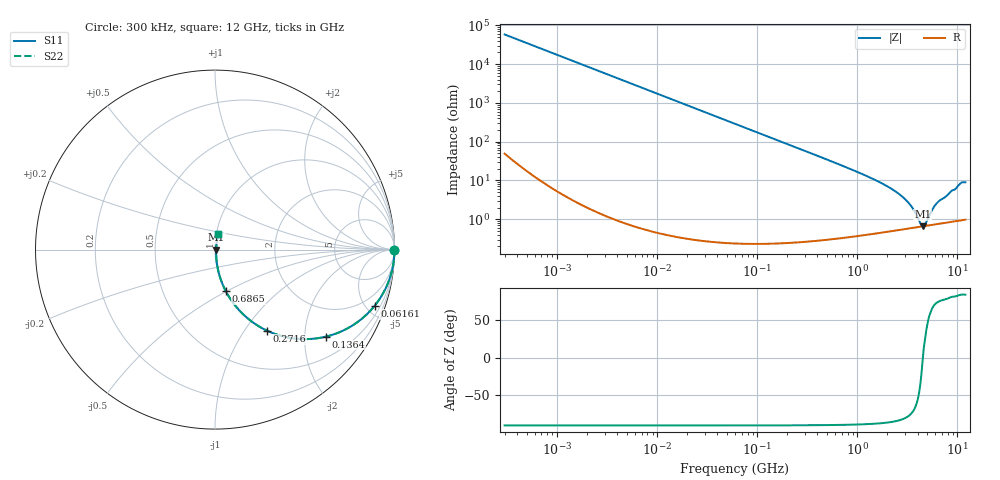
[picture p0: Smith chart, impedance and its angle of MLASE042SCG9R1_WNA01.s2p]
! MLASE042SCG9R1_WNA01  S-PARAMETER MODEL  ( General Type )
! Model Generated by TAIYO YUDEN Corporation (http://www.ty-top.com)
! Version 1.0
! TAIYO YUDEN Control No. 130801
! Copyright(c) 2013 TAIYO YUDEN CO.,LTD. All Rights Reserved.
! Product Description (link to TY-COMPAS)
! https://ds.yuden.co.jp/TYCOMPAS/or/detail?pn=MLASE042SCG9R1BWNA01&u=M
! Products Name : Multilayer Ceramic Capacitors
! Characteristics :
!  Capacitance : 9.1 pF , Rated Voltage : 16V , TCC : CG / C0G
!  Case Size : 0.4 x 0.2 / 0.016 x 0.008 [mm/inch] , Thickness : 0.2 / 0.008 [mm/inch]
!  (Conditions: Temperature = 25 degC , DC Bias Current/Voltage = 0A / 0V)
! External Node Assignments :
!  1  o---| |---o  2
! GND o---------o GND
! Frequency Range : 0.3MHz  -  12000MHz  [ 401 STEP ]
# MHz S RI R 50
! Freq[MHz].  S11 Real  S11 Imag  S21 Real  S21 Imag  S12 Real  S12 Imag  S22 Real  S22 Imag
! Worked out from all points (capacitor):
!   401 points, 300 kHz to 12 GHz, reference 50 ohm
!   read as one part in series: C = 9.13 pF near 316.3 kHz
!   lowest |Z| = 659 mohm at 4.503 GHz (marker M1)
!   series resonance near 4.513 GHz, so ESL is about 140 pH
!   S11 on the Smith chart (normalised r, x): 300 kHz: open; 61.61 MHz: 1.00, -5.66; 136.4 MHz: 1.00, -2.55; 271.6 MHz: 1.01, -1.28; 686.5 MHz: 1.01, -0.50; 12 GHz: 1.02, +0.18
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0.3  1 -0.00172  4.41e-06 0.00172  4.41e-06 0.00172  1 -0.00172
1.769972  0.9999 -0.0101  0.000105 0.0101  0.000105 0.0101  0.9999 -0.0101
10.44266  0.9964 -0.0597  0.00359 0.0597  0.00359 0.0597  0.9964 -0.0597
26.39317  0.9775 -0.148  0.0225 0.148  0.0225 0.148  0.9775 -0.148
60  0.8939 -0.3076  0.1061 0.3076  0.1061 0.3076  0.8939 -0.3076
61.61074  0.8888 -0.314  0.1112 0.314  0.1112 0.314  0.8888 -0.314
136.3989  0.6198 -0.4845  0.3802 0.4845  0.3802 0.4845  0.6198 -0.4845
271.6094  0.2911 -0.4523  0.7089 0.4523  0.7089 0.4523  0.2911 -0.4523
353.9943  0.1947 -0.3932  0.8053 0.3932  0.8053 0.3932  0.1947 -0.3932
686.4755  0.0607 -0.2323  0.9393 0.2323  0.9393 0.2323  0.0607 -0.2323
1331.232  0.018 -0.117  0.982 0.117  0.982 0.117  0.018 -0.117
2088.533  0.00904 -0.0647  0.991 0.0647  0.991 0.0647  0.00904 -0.0647
2650.866  0.00711 -0.0426  0.9929 0.0426  0.9929 0.0426  0.00711 -0.0426
3190.978  0.00643 -0.027  0.9936 0.027  0.9936 0.027  0.00643 -0.027
3642.919  0.00628 -0.0165  0.9937 0.0165  0.9937 0.0165  0.00628 -0.0165
4270.516  0.00642 -0.00424  0.9936 0.00424  0.9936 0.00424  0.00642 -0.00424
4502.883  0.00655 -0.000145  0.9935 0.000145  0.9935 0.000145  0.00655 -0.000145
4747.894  0.0067 0.00309  0.9933 -0.00309  0.9933 -0.00309  0.0067 0.00309
5715.274  0.00752 0.0175  0.9925 -0.0175  0.9925 -0.0175  0.00752 0.0175
6354.153  0.00821 0.026  0.9918 -0.026  0.9918 -0.026  0.00821 0.026
10793.46  0.0162 0.0827  0.9838 -0.0827  0.9838 -0.0827  0.0162 0.0827
12000  0.0173 0.0867  0.9827 -0.0867  0.9827 -0.0867  0.0173 0.0867
